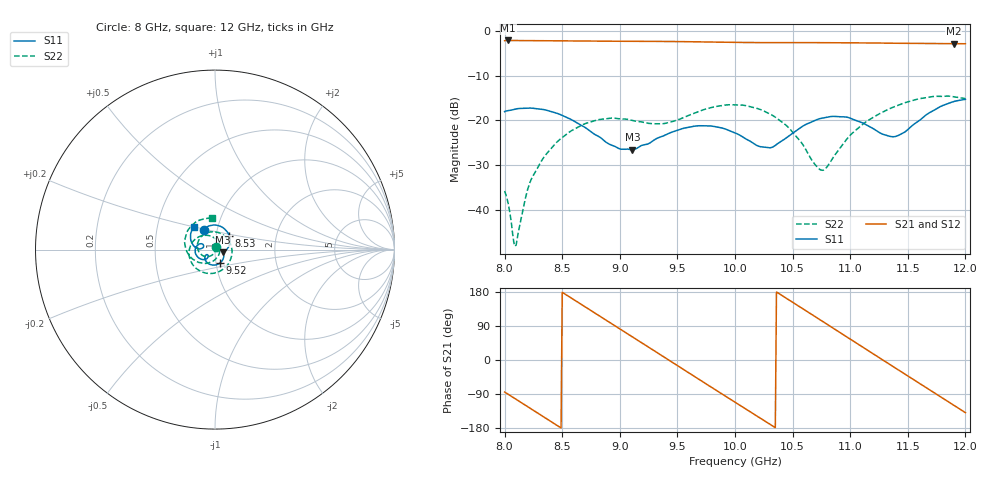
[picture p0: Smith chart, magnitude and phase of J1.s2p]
!Keysight Technologies,N5234A,MY52241180,A.10.60.03
!Date: Tuesday, May 30, 2023 15:16:02
!Correction: S11(Full 2 Port(1,2))
!S21(Full 2 Port(1,2))
!S12(Full 2 Port(1,2))
!S22(Full 2 Port(1,2))
!S2P File: Measurements: S11, S21, S12, S22:
# Hz S  dB  R 50
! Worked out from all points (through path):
!   401 points, 8 GHz to 12 GHz, reference 50 ohm
!   highest |S21| = -2.13 dB at 8.03 GHz (marker M1); lowest = -2.9 dB at 11.9 GHz (marker M2)
!   group delay of S21, straight-line fit = 538 ps
!   lowest |S11| = -26.6 dB at 9.11 GHz (marker M3), VSWR 1.10, Z = 54.7 - j1.58 ohm
!   |S11| at or under -10 dB: start of sweep to end of sweep
!   |S22| runs from -48.1 to -14.6 dB; largest |S21 - S12| = 0.0014
!   S11 on the Smith chart (normalised r, x): 8 GHz: 0.87, +0.19; 8.53 GHz: 1.16, +0.18; 9.52 GHz: 1.05, -0.16; 12 GHz: 0.77, +0.20
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8e9  -18.03 118.3  -2.19 -84.5  -2.19 -84.5  -35.75 67.5
8.03e9  -17.82 115.6  -2.13 -90.2  -2.14 -90.2  -38.42 60.6
8.1e9  -17.43 107.8  -2.15 -103.8  -2.15 -103.8  -47.84 -41.6
8.24e9  -17.26 88.9  -2.16 -130.9  -2.17 -131.0  -32.69 -110.1
8.53e9  -19.22 43.3  -2.21 172.9  -2.22 172.9  -23.23 -146.7
8.67e9  -21.15 21.6  -2.24 145.8  -2.25 145.8  -21.06 -168.6
8.9e9  -25.20 -7.1  -2.29 101.5  -2.31 101.5  -19.57 147.6
9.11e9  -26.55 -17.9  -2.32 61.0  -2.33 60.9  -20.00 97.9
9.34e9  -23.82 -41.2  -2.35 16.4  -2.36 16.3  -20.77 26.1
9.52e9  -22.03 -69.1  -2.39 -18.6  -2.40 -18.6  -19.72 -35.1
9.77e9  -21.21 -110.1  -2.48 -67.1  -2.49 -67.1  -17.28 -103.3
1e10  -22.78 -141.0  -2.56 -111.3  -2.57 -111.4  -16.53 -154.5
1.034e10  -25.75 -135.5  -2.62 -176.7  -2.62 -176.7  -19.09 137.8
1.05e10  -22.85 -133.8  -2.61 152.4  -2.62 152.4  -22.64 102.9
1.067e10  -20.28 -148.2  -2.61 119.4  -2.62 119.4  -28.96 46.8
1.078e10  -19.36 -161.9  -2.62 98.1  -2.63 98.0  -30.90 -22.6
1.096e10  -19.22 176.2  -2.64 63.0  -2.65 63.0  -24.52 -93.4
1.116e10  -21.26 157.7  -2.69 24.0  -2.69 24.0  -19.93 -131.4
1.134e10  -23.53 161.8  -2.73 -11.0  -2.74 -11.0  -17.40 -157.0
1.164e10  -19.16 173.4  -2.82 -69.2  -2.83 -69.3  -15.00 158.7
1.19e10  -15.77 145.9  -2.87 -119.5  -2.87 -119.6  -14.71 114.8
1.2e10  -15.28 133.1  -2.87 -138.9  -2.88 -138.9  -15.15 95.3
